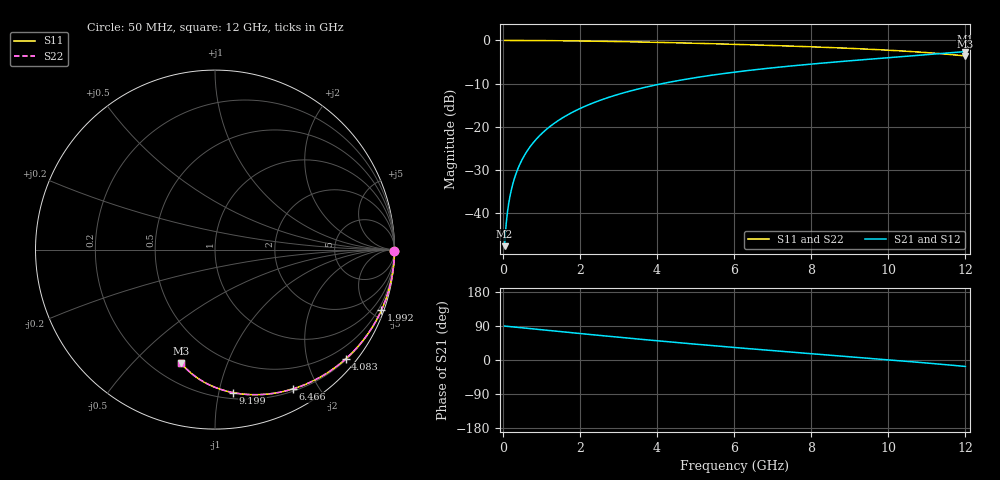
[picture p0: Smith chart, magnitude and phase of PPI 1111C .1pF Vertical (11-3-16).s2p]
# GHz S MA R 50
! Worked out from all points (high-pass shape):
!   1601 points, 50 MHz to 12 GHz, reference 50 ohm
!   highest |S21| = -2.58 dB at 12 GHz (marker M1); lowest = -47.7 dB at 50 MHz (marker M2)
!   |S21| within 3 dB of the highest: 7.873 GHz to end of sweep
!   lowest |S11| = -3.6 dB at 12 GHz (marker M3), VSWR 4.90, Z = 15.5 - j35 ohm
!   |S11| at or under -10 dB: nowhere
!   |S22| runs from -3.6 to 0.0 dB; largest |S21 - S12| = 0
!   S11 on the Smith chart (normalised r, x): 50 MHz: open; 1.992 GHz: 0.22, -5.66; 4.083 GHz: 0.22, -2.74; 6.466 GHz: 0.23, -1.69; 9.199 GHz: 0.25, -1.10; 12 GHz: 0.31, -0.70
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0.05  1 -0.5  0.004144 89.5  0.004144 89.5  1 -0.5
0.1545625  0.9999 -1.6  0.01281 88.4  0.01281 88.4  0.9999 -1.6
0.1919063  0.9999 -1.9  0.0159 88.1  0.0159 88.1  0.9999 -1.9
0.2441875  0.9998 -2.5  0.02023 87.5  0.02023 87.5  0.9998 -2.5
0.378625  0.9995 -3.8  0.03136 86.2  0.03136 86.2  0.9995 -3.8
0.5653438  0.9989 -5.7  0.04677 84.3  0.04677 84.3  0.9989 -5.7
0.8192812  0.9977 -8.3  0.06766 81.7  0.06766 81.7  0.9977 -8.3
1.132969  0.9956 -11.5  0.09326 78.5  0.09326 78.5  0.9956 -11.5
1.521344  0.9921 -15.3  0.1246 74.6  0.1246 74.6  0.9921 -15.3
1.991875  0.9867 -20.0  0.1617 70.0  0.1617 70.0  0.9867 -20.0
2.044156  0.986 -20.5  0.1658 69.5  0.1658 69.5  0.986 -20.5
2.932937  0.9722 -29.1  0.2328 60.8  0.2328 60.8  0.9722 -29.1
4.038312  0.9503 -39.5  0.3098 50.4  0.3098 50.4  0.9503 -39.5
4.083125  0.9493 -39.9  0.3128 50.0  0.3128 50.0  0.9493 -39.9
5.046594  0.9268 -48.5  0.3736 41.4  0.3736 41.4  0.9268 -48.5
6.025  0.9017 -57.0  0.4301 32.9  0.4301 32.9  0.9017 -57.0
6.465656  0.8897 -60.7  0.454 29.2  0.454 29.2  0.8897 -60.7
8.019156  0.8438 -73.3  0.5333 16.5  0.5333 16.5  0.8438 -73.3
9.199219  0.8034 -82.7  0.5912 7.0  0.5912 7.0  0.8034 -82.7
10.01331  0.771 -89.3  0.632 0.4  0.632 0.4  0.771 -89.3
11.01412  0.7227 -97.7  0.6852 -8.1  0.6852 -8.1  0.7227 -97.7
12  0.6609 -106.5  0.7431 -17.1  0.7431 -17.1  0.6609 -106.5
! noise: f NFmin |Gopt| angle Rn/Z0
0.05  0.006459  0.9959  0.5067  0.3589
1.372  0.007857  0.8949  12.62  0.01612
2.701  0.009846  0.8168  22.12  0.01084
4.031  0.012  0.7626  29.85  0.009587
5.36  0.01426  0.7269  36.52  0.009389
6.682  0.01664  0.7052  42.42  0.009678
8.012  0.01923  0.694  47.81  0.01031
9.341  0.02209  0.6914  52.77  0.01128
10.67  0.02531  0.6958  57.36  0.01262
12  0.02901  0.7062  61.67  0.01445
